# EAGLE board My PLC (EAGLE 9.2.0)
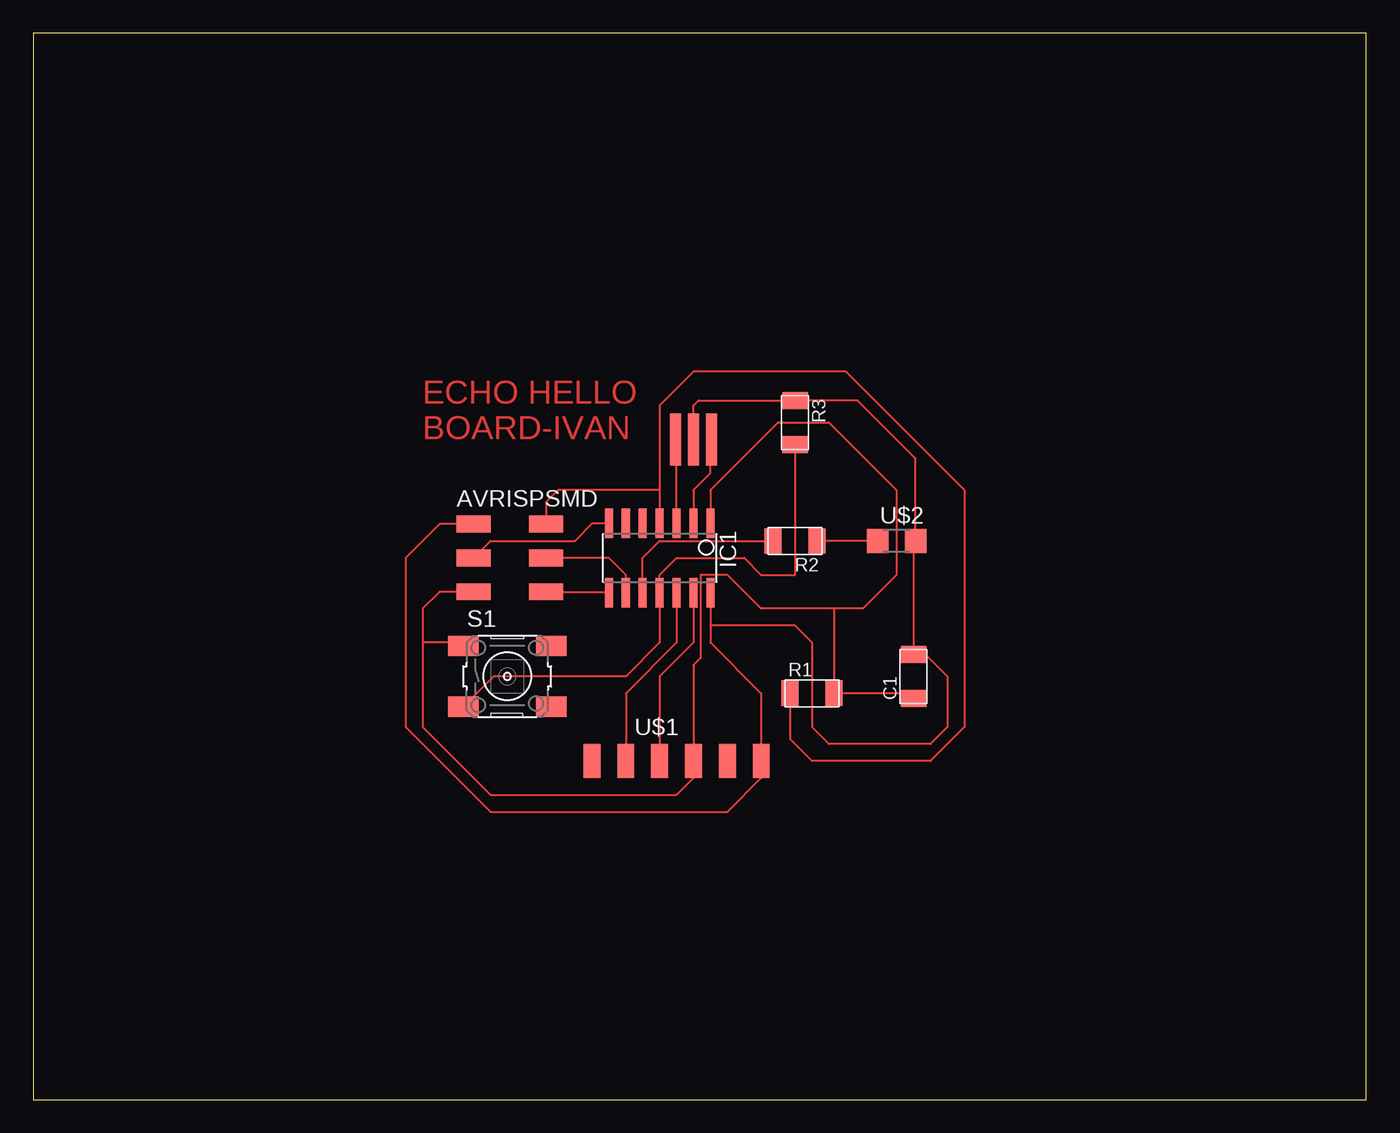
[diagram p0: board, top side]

Size 100 x 80 mm. Coordinates in mm from the lower left corner, seen from the top.
Outline: 0,0 100,0 100,80 0,80 0,0
Copper layers (1*16): Top 0.035mm / dielectric 1.5mm / Bottom 0.035mm
Design rules "default": minimum track width 6mil, minimum drill 0.35mm, track to track 6mil, track to pad 6mil, pad to pad 6mil, via to via 6mil, smd to smd 6mil, copper to edge 40mil, drill to drill 6mil, minimum pad ring 10mil, minimum via ring 8mil, stop-mask expansion 4mil, vias tented up to drill 0mil, thermal gap 10mil

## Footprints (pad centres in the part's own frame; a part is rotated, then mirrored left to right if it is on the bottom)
2X03SMD = smd 2.54 x 1.27: 1 -2.54,2.54; 2 2.92,2.54; 3 -2.54,0; 4 2.92,0; 5 -2.54,-2.54; 6 2.92,-2.54
C1206FAB = smd 1.27 x 1.905: 1 -1.651,0; 2 1.651,0
SOIC14 = smd 0.61 x 2.21: 1 -3.81,-2.603; 2 -2.54,-2.603; 3 -1.27,-2.603; 4 0,-2.603; 5 1.27,-2.603; 6 2.54,-2.603; 7 3.81,-2.603; 8 3.81,2.603; 9 2.54,2.603; 10 1.27,2.603; 11 0,2.603; 12 -1.27,2.603; 13 -2.54,2.603; 14 -3.81,2.603
R1206FAB = smd 1.27 x 1.905: 1 -1.651,0; 2 1.651,0
6MM_SWITCH = smd 2.286 x 1.524: 1 -3.302,2.286; 2 3.302,2.286; 3 -3.302,-2.286; 4 3.302,-2.286
1X06SMD = smd 2.54 x 1.27: 1 0,6.35; 2 0,3.81; 3 0,1.27; 4 0,-1.27; 5 0,-3.81; 6 0,-6.35
LED1206 = smd 1.6 x 1.803: 1 -1.422,0; 2 1.422,0
EFOBM = smd 0.8 x 3.9: 1 -1.35,0; 2 0,0; 3 1.35,0

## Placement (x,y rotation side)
AVRISPSMD  [2X03SMD]  35.56,40.64 0 top
C1  1uF  [C1206FAB]  66.04,31.75 90 top
IC1  UC_ATTINY44-SSU  [SOIC14]  46.99,40.64 180 top
R1  10kΩ  [R1206FAB]  58.42,30.48 0 top
R2  499Ω  [R1206FAB]  57.15,41.91 180 top
R3  499Ω  [R1206FAB]  57.15,50.8 270 top
S1  [6MM_SWITCH]  35.56,31.75 0 top
U$1  CONN_06_FTDI-SMD-HEADER  [1X06SMD]  48.26,25.4 270 top
U$2  LED  [LED1206]  64.77,41.91 0 top
U$3  XTAL_RESONATOR  [EFOBM]  49.53,49.53 180 top

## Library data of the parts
AVRISPSMD C1 IC1 R1-R3 S1 U$1-U$3 = fab

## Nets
GND: AVRISPSMD.1 C1.2 IC1.14 R3.1 U$1.1 U$2.2 U$3.2
MISO: AVRISPSMD.6 IC1.8
MOSI: AVRISPSMD.3 IC1.7
N$3: IC1.11 R3.2 S1.3
N$6: IC1.10 R2.2
N$9: IC1.2 U$3.1
N$10: IC1.3 U$3.3
N$13: R2.1 U$2.1
RST: AVRISPSMD.2 IC1.4 R1.1
RXD: IC1.12 U$1.5
SCK: AVRISPSMD.4 IC1.9
TXD: IC1.13 U$1.4
VCC: AVRISPSMD.5 C1.1 IC1.1 R1.2 S1.1 U$1.3

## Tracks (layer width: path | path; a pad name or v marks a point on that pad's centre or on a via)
GND
  Top 0.152: AVRISPSMD.1 30.48,43.18 27.94,40.64 27.94,27.94 34.29,21.59 52.07,21.59 54.61,24.13 U$1.1 54.61,30.48 50.8,34.29 IC1.14 50.8,35.56 57.15,35.56 58.42,34.29 58.42,27.94 59.69,26.67 67.31,26.67 68.58,27.94 68.58,31.75 66.93,33.4 C1.2 66.04,41.76 U$2.2 66.19,48.11 61.85,52.45 R3.1 | U$3.2 49.53,52.07 49.91,52.45 R3.1 | R3.1 57.15,52.07
MISO
  Top 0.152: IC1.8 38.54,38.04 AVRISPSMD.6
MOSI
  Top 0.152: AVRISPSMD.3 34.29,41.91 40.64,41.91 41.97,43.24 IC1.7
N$3
  Top 0.152: S1.3 34.54,31.75 44.45,31.75 46.99,34.29 IC1.11 46.99,39.37 48.26,40.64 53.34,40.64 54.61,39.37 57.15,39.37 R3.2
N$6
  Top 0.152: IC1.10 45.72,40.64 46.99,41.91 R2.2
N$9
  Top 0.152: IC1.2 49.53,45.72 50.8,46.99 50.8,49.45 U$3.1
N$10
  Top 0.152: IC1.3 48.26,49.45 U$3.3
N$13
  Top 0.152: U$2.1 R2.1
RST
  Top 0.152: 46.99,45.72 39.37,45.72 38.48,44.83 AVRISPSMD.2 | 46.99,45.72 IC1.4 | R1.1 56.77,27.05 58.42,25.4 67.31,25.4 69.85,27.94 69.85,45.72 60.96,54.61 49.53,54.61 46.99,52.07 46.99,45.72
RXD
  Top 0.152: IC1.12 48.26,34.29 44.45,30.48 U$1.5
SCK
  Top 0.152: IC1.9 44.45,39.37 43.18,40.64 AVRISPSMD.4
TXD
  Top 0.152: U$1.4 46.99,31.75 49.53,34.29 IC1.13
VCC
  Top 0.152: 29.21,34.29 29.21,27.94 34.29,22.86 48.26,22.86 49.53,24.13 U$1.3 49.53,32.59 50.06,33.12 50.06,39.37 52.07,39.37 54.61,36.83 60.07,36.83 | AVRISPSMD.5 30.48,38.1 29.21,36.83 29.21,34.29 | S1.1 32,34.29 29.21,34.29 | C1.1 65.66,30.48 R1.2 60.07,36.83 | 60.07,36.83 62.23,36.83 64.77,39.37 64.77,45.72 59.69,50.8 55.88,50.8 50.8,45.72 IC1.1

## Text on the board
Top: ECHO HELLO / BOARD-IVAN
